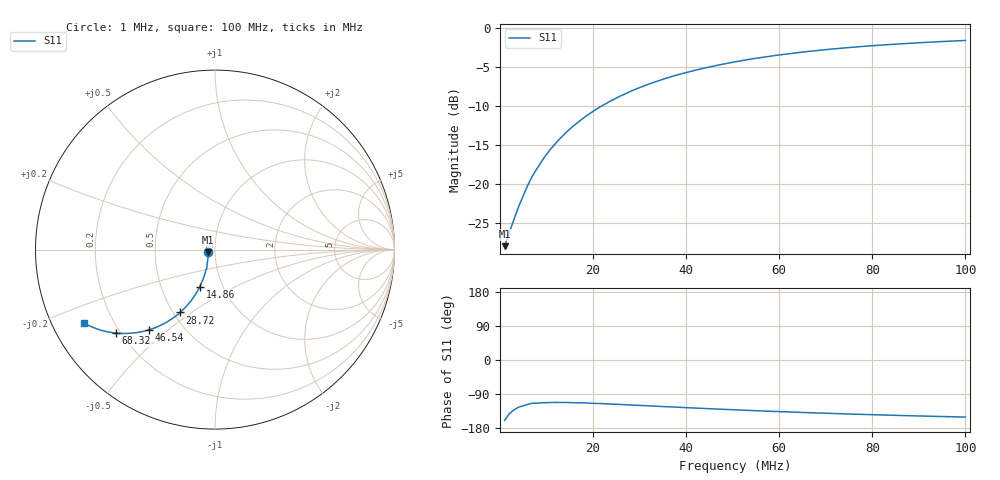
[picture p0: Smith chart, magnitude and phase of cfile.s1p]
# Hz S RI R 50.0
! written by SimSmith version 18.3b
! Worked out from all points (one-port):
!   101 points, 1 MHz to 100 MHz, reference 50 ohm
!   lowest |S11| = -28.0 dB at 1 MHz (marker M1), VSWR 1.08, Z = 46.4 - j1.31 ohm
!   |S11| at or under -10 dB: start of sweep to 21.82 MHz
!   S11 on the Smith chart (normalised r, x): 1 MHz: 0.93, -0.03; 14.86 MHz: 0.78, -0.34; 28.72 MHz: 0.54, -0.45; 46.54 MHz: 0.32, -0.43; 68.32 MHz: 0.18, -0.35; 100 MHz: 0.10, -0.26
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1000000  -0.037 -0.014
1990000  -0.0381 -0.0297
3970000  -0.0402 -0.0581
5950000  -0.0445 -0.0865
6940000  -0.0454 -0.1019
7930000  -0.051 -0.1138
9910000  -0.0587 -0.1418
1.09e7  -0.063 -0.155
1.189e7  -0.0678 -0.1677
1.387e7  -0.0783 -0.1935
1.486e7  -0.0842 -0.2061
1.783e7  -0.1039 -0.242
1.981e7  -0.1188 -0.2642
2.179e7  -0.1334 -0.2863
2.575e7  -0.1675 -0.325
2.872e7  -0.1947 -0.3504
3.367e7  -0.2414 -0.3869
3.862e7  -0.2895 -0.4156
4.357e7  -0.3376 -0.4371
4.654e7  -0.3659 -0.4465
5.05e7  -0.4028 -0.4566
5.644e7  -0.4561 -0.4648
6.337e7  -0.5136 -0.467
6.832e7  -0.5515 -0.4644
7.525e7  -0.5989 -0.4581
8.119e7  -0.6353 -0.4493
8.812e7  -0.6733 -0.4358
1e8  -0.7286 -0.4103
